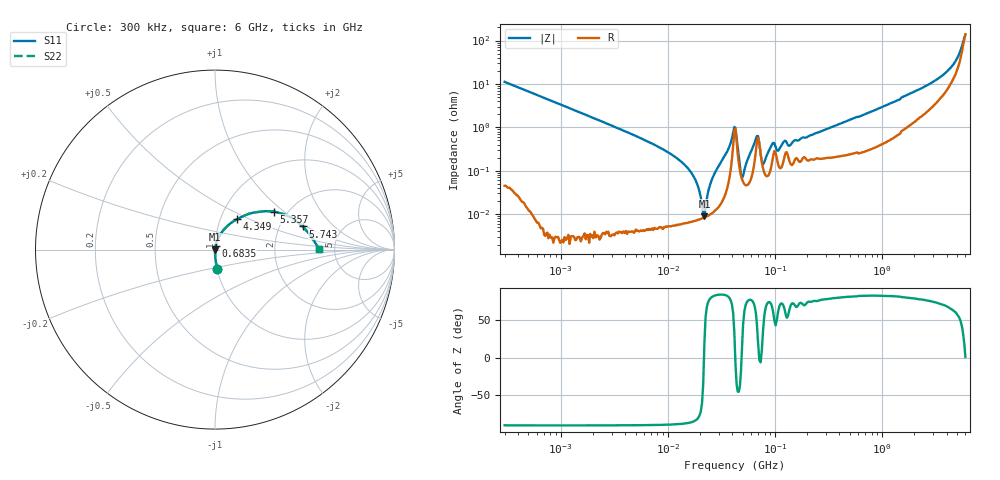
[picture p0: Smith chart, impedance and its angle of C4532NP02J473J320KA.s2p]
! S-Parameter Data Generated by TDK Corporation
! Copyright(C) 2024 TDK Corporation.
! All Rights Reserved.
! TDK P/N: C4532NP02J473J320KA (Multilayer Ceramic Chip Capacitor)
! Property: C=47nF
! Size(LxWxT): 4.5x3.2x3.2mm
! Model Type: s2p (Touchstone File Format Version 1.0)
! Frequency: DC=Yes Start=0.3MHz Stop=6000MHz 402points Log-sweep
! Model Generated on May 28, 2024
! Terms and conditions regarding TDK Simulation Models:
! 1)This simulation model is being provided solely for informational
!  purposes. Please refer to the specifications of the products in
!  terms of detailed characteristics of such products.
! 2)In no event shall TDK Corporation of any of its subsidiaries be
!  liable for any loss or damage arising, directly or indirectly,
!  from any information contained in this simulation model, including,
!  but not limited to loss or damages arising from any inaccuracies,
!  omissions or errors in connection with such information.
! 3)Any and all copyrights on this simulation model are owned by
!  TDK Corporation.  Duplication or redistribution of this simulation
!  model without prior written permission from TDK Corporation
!  is prohibited.
! 4)This simulation model is subject to any modification or change
!  without any prior notice.
! 5)Neither TDK Corporation nor any of its subsidiaries shall make any
!  warranty, express or implied, including but not limited to the
!  correctness, implied warranties of merchantability and fitness for
!  a particular purpose with respect to this simulation models.
! 6)The use of this simulation model shall be deemed to have consented
!  to the terms and conditions hereof.
! Port Assignments:
!  1 ---| |--- 2
! Applicable Conditions:
!  Temperature = 25 degC
!  DC Bias Voltage = 0 V
!  Small Signal Operation
# Hz S MA R 50
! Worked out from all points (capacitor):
!   401 points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, 300 kHz to 6 GHz, reference 50 ohm
!   read as one part in series: C = 47.4 nF near 317.3 kHz
!   lowest |Z| = 8.92 mohm at 21.98 MHz (marker M1)
!   series resonance near 21.79 MHz, so ESL is about 1.1 nH
!   S11 on the Smith chart (normalised r, x): 300 kHz: 1.00, -0.22; 683.5 MHz: 1.01, +0.04; 4.349 GHz: 1.20, +0.42; 5.357 GHz: 1.71, +0.86; 5.743 GHz: 2.68, +0.93; 6 GHz: 3.76, +0.04
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300000  0.1111 -83.4  0.9934 6.4  0.9934 6.4  0.1111 -83.4
1586297  0.02104 -88.7  0.9997 1.2  0.9997 1.2  0.02104 -88.7
8158352  0.003571 -89.0  0.9999 0.2  0.9999 0.2  0.003571 -89.0
1.593136e7  0.00103 -86.3  0.9999 0.1  0.9999 0.1  0.00103 -86.3
1.833994e7  0.0005753 -82.9  0.9999 0.0  0.9999 0.0  0.0005753 -82.9
2.198043e7  8.923e-05 19.6  0.9999 -0.0  0.9999 -0.0  8.923e-05 19.6
2.650558e7  0.0007346 81.4  0.9999 -0.0  0.9999 -0.0  0.0007346 81.4
3.49112e7  0.002447 82.5  0.9997 -0.1  0.9997 -0.1  0.002447 82.5
4.078682e7  0.007502 58.6  0.9961 -0.4  0.9961 -0.4  0.007502 58.6
4.28954e7  0.009371 -9.6  0.9908 0.1  0.9908 0.1  0.009371 -9.6
4.922114e7  0.0006631 11.2  0.9993 -0.0  0.9993 -0.0  0.0006631 11.2
6.645562e7  0.005456 58.7  0.9972 -0.3  0.9972 -0.3  0.005456 58.7
7.964712e7  0.00159 55.5  0.9991 -0.1  0.9991 -0.1  0.00159 55.5
9.369548e7  0.003987 68.3  0.9985 -0.2  0.9985 -0.2  0.003987 68.3
1.071199e8  0.002893 60.8  0.9986 -0.1  0.9986 -0.1  0.002893 60.8
2.249926e8  0.006799 74.2  0.9982 -0.4  0.9982 -0.4  0.006799 74.2
6.835422e8  0.01973 80.9  0.9971 -1.1  0.9971 -1.1  0.01973 80.9
1.174439e9  0.03453 79.8  0.9944 -2.0  0.9944 -2.0  0.03453 79.8
4.348783e9  0.2082 54.1  0.8938 -10.9  0.8938 -10.9  0.2082 54.1
5.357416e9  0.3922 32.8  0.703 -17.6  0.703 -17.6  0.3922 32.8
5.742966e9  0.5059 14.8  0.5269 -14.2  0.5269 -14.2  0.5059 14.8
6e9  0.5798 0.4  0.4202 -0.5  0.4202 -0.5  0.5798 0.4
